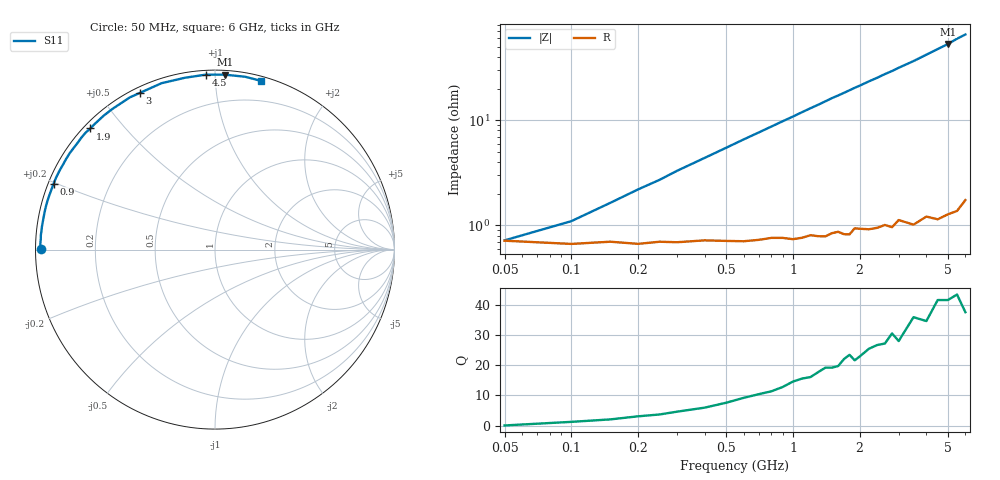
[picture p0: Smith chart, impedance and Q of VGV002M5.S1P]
! Infineon Technologies  Discrete & RF Semiconductors
! BB 831
! Si Tuning Diode in SOD323
! VR =
! S-Parameters:  July  1999
# GHz  S  MA  R  50
!  f  S11
! GHz  MAG  ANG
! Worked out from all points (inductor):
!   34 points, 50 MHz to 6 GHz, reference 50 ohm
!   read as one part to ground: L = 1.67 nH near 200 MHz
!   highest Q = 41.5 at 5 GHz (marker M1), where L = 1.68 nH
!   S11 on the Smith chart (normalised r, x): 50 MHz: 0.01, +0.00; 900 MHz: 0.02, +0.20; 1.9 GHz: 0.02, +0.41; 3 GHz: 0.02, +0.63; 4.5 GHz: 0.02, +0.95; 6 GHz: 0.03, +1.30
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0.05  0.9718 179.8
0.1  0.9737 178.0
0.2  0.9737 175.2
0.25  0.9725 174.0
0.3  0.9728 172.6
0.5  0.9722 167.6
0.6  0.9725 165.1
0.8  0.9708 160.3
0.9  0.9711 157.9
1  0.9721 155.6
1.1  0.9715 153.2
1.4  0.9715 146.4
1.5  0.9699 144.1
1.6  0.9693 142.1
1.8  0.9718 137.9
1.9  0.9683 135.8
2  0.969 133.9
2.2  0.9702 129.9
2.4  0.9702 126.3
2.6  0.9694 122.5
2.8  0.9718 119.2
3  0.9683 115.6
3.5  0.9738 107.8
4  0.9719 100.0
4.5  0.9762 93.0
5  0.9762 86.8
5.5  0.9775 80.1
6  0.9746 74.9
